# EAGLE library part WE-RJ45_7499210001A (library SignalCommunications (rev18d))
Order Code 7499210001A Design THT xBase-T 10/100 Base-T PoE Ports 1x1 Application PoE Tab Position UP LED (Left-Right) NONE EMI Fingers No Details see: http://katalog.we-online.de/en/pbs/WE-LAN_RJ45/7499210001A? Updated by Yingchun Shan 2016-08-30 2016(C) Würth Elektronik
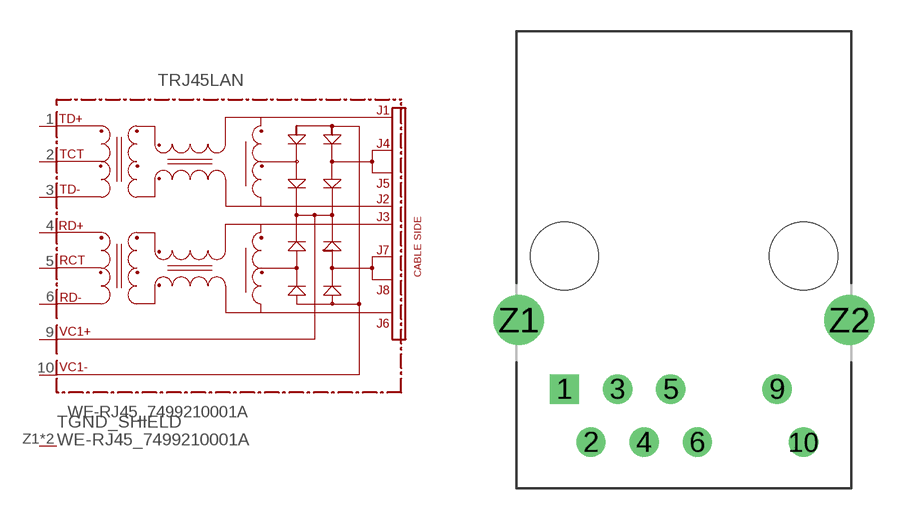
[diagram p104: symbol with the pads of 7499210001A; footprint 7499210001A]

Designator prefix T; gates RJ45LAN=749921-THT-POE-RVS GND_SHIELD=GND_PIN

## WE-RJ45_7499210001A (COMPANY-URL: http://www.we-online.de; CREATED-BY: Christin Zierenner; CREATED-DATE: AUG 2012; DATASHEET-URL: http://katalog.we-online.de/kataloge/eisos/media/pdf/7499210001A.pdf; MANUFACTURER: Würth Elektronik eiSos GmbH)  [7499210001A]
1  RJ45LAN:TD+
2  RJ45LAN:TCT
3  RJ45LAN:TD-
4  RJ45LAN:RD+
5  RJ45LAN:RCT
6  RJ45LAN:RD-
9  RJ45LAN:VC1+  pwr
10  RJ45LAN:VC1-  pwr
Z1  GND_SHIELD:1  pwr
Z2  GND_SHIELD:1  pwr

## Footprint 7499210001A (pad centres in mm)
MAX HEIGHT=13.74mm PORTS----1X1 LED --NO
drill 0.89 square: 1 -5.715,-6.35
drill 0.89: 2 -4.445,-8.89; 3 -3.175,-6.35; 4 -1.905,-8.89; 5 -0.635,-6.35; 6 0.635,-8.89; 9 4.445,-6.35; 10 5.715,-8.89
drill 1.6: Z1 -7.9,-3.05; Z2 7.9,-3.05
hole 3.25 at 5.715,0
hole 3.25 at -5.715,0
